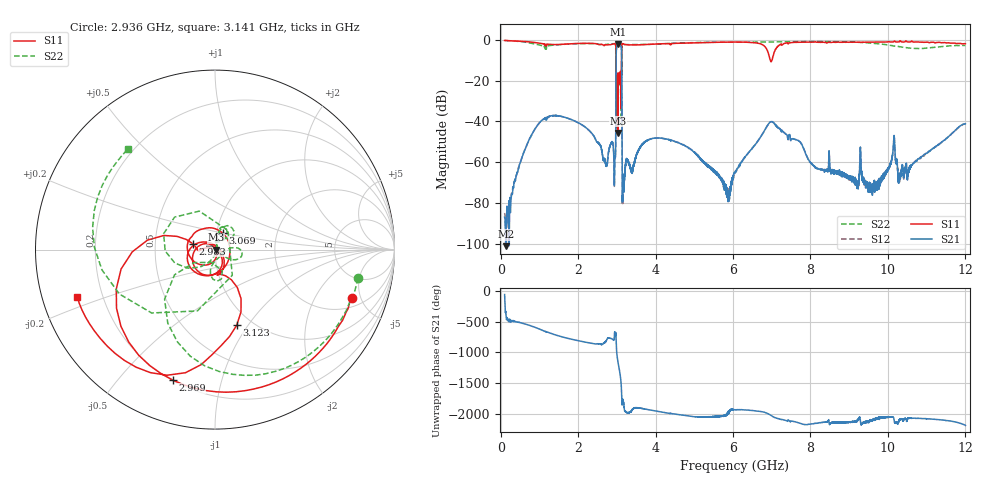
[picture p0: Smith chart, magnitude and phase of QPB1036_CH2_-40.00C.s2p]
! TDS: K:\Engsetup\Winsaw\QPB1036_ALL
! Channel 1
! Ports=1 2
! seg 1=100.000000 1100.000000 101
! seg 2=1101.000000 1501.000000 401
! seg 3=1502.000000 2502.000000 101
! seg 4=2503.000000 3803.000000 1301
! seg 5=3804.000000 5004.000000 121
! seg 6=5005.000000 6005.000000 1001
! seg 7=6006.000000 8406.000000 241
! seg 8=8407.000000 10607.000000 2201
! seg 9=10608.000000 12008.000000 141
! Points=5609
! FailCode=0
! Topology=ALL_SE(12)
!VNA Cal loaded =QPB1036_ALL_-40C
!PS1(V)= 5.000
!PS(mA)= 0.500
!PS2(V)= 0.630
!PS(mA)= -0.100
!PS3(V)= 1.170
!PS(mA)= 0.100
!PS4(V)= 0.630
!PS(mA)= -0.100
!Temp (C)= -40.00
# MHz S DB R 50
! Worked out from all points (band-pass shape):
!   5609 points, 100 MHz to 12.01 GHz, reference 50 ohm
!   highest |S21| = -2.11 dB at 3.036 GHz (marker M1); lowest = -101.2 dB at 130 MHz (marker M2)
!   |S21| within 3 dB of the highest: 2.987 GHz to 3.121 GHz (134 MHz wide, 4.39 % of centre)
!   lowest |S11| = -45.6 dB at 3.027 GHz (marker M3), VSWR 1.01, Z = 50.5 - j0.0251 ohm
!   |S11| at or under -10 dB: 2.98 GHz to 3.121 GHz (141.4 MHz wide, 4.63 % of centre); 6.969 GHz to 7.006 GHz (36.96 MHz wide, 0.529 % of centre)
!   |S22| runs from -39.3 to -0.3 dB; largest |S21 - S12| = 0.0068
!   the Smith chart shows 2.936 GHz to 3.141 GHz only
!   S11 on the Smith chart (normalised r, x): 2.936 GHz: 2.69, -4.15; 2.969 GHz: 0.20, -0.71; 2.983 GHz: 0.78, +0.05; 3.069 GHz: 1.07, +0.20; 3.123 GHz: 0.85, -0.89; 3.141 GHz: 0.11, -0.16
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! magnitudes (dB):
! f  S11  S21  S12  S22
! 100 MHz  -0.2  -87.0  -84.9  -0.3
! 130 MHz  -0.3  -101.2  -88.1  -0.3
! 1.124 GHz  -2.0  -38.9  -38.8  -3.3
! 2.092 GHz  -1.7  -41.6  -41.6  -1.8
! 2.936 GHz  -1.9  -71.4  -71.9  -1.8
! 2.969 GHz  -2.3  -53.4  -53.4  -3.1
! 2.983 GHz  -17.8  -7.2  -7.2  -16.8
! 3.027 GHz  -45.6  -2.2  -2.2  -24.6
! 3.036 GHz  -21.6  -2.1  -2.1  -31.4
! 3.069 GHz  -19.9  -2.3  -2.3  -17.6
! 3.102 GHz  -22.0  -2.9  -2.8  -19.7
! 3.123 GHz  -7.2  -6.3  -6.3  -10.5
! 3.141 GHz  -1.8  -71.6  -69.7  -2.6
! 3.167 GHz  -1.9  -66.0  -67.7  -2.3
! 4.074 GHz  -1.9  -48.2  -48.0  -2.0
! 5.881 GHz  -1.1  -79.1  -77.2  -1.1
! 6.056 GHz  -1.0  -64.8  -65.2  -1.1
! 7.026 GHz  -8.8  -40.2  -40.2  -0.9
! 8.046 GHz  -1.1  -61.1  -60.9  -0.7
! 10.02 GHz  -0.8  -63.0  -62.6  -2.5
! 10.16 GHz  -0.7  -47.8  -47.8  -3.0
! 12.01 GHz  -1.8  -41.2  -41.1  -2.7
